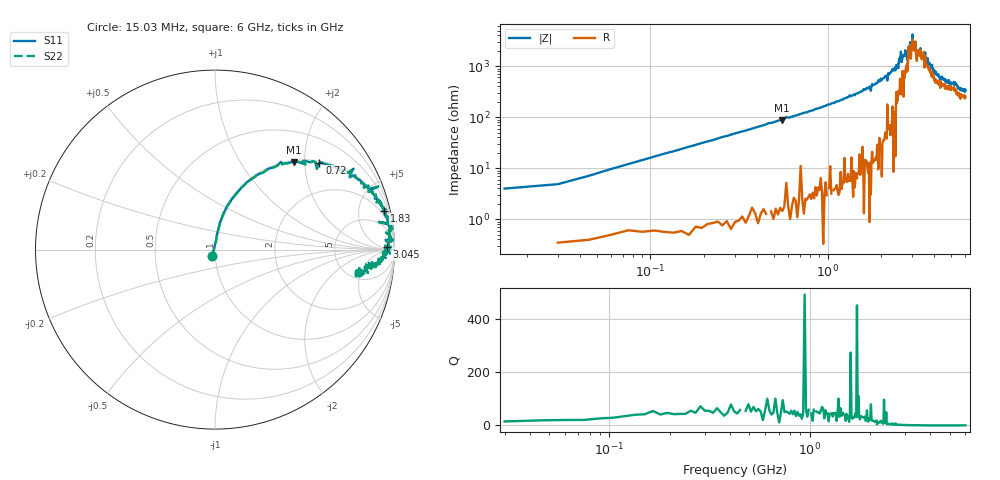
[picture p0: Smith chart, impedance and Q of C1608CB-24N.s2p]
!	Network	Analyzer	HP8753E.07.74:	Oct	30	2002	Serial	No.	JP38451487
!	Hewlett-Packard
!	28	Aug	2009	16:01:57
!	Frequency	S11	S21	S12	S22
#	HZ	S	RI	R	50
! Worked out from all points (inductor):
!   400 points, 15.03 MHz to 6 GHz, reference 50 ohm
!   read as one part in series: L = 25.5 nH near 45.03 MHz
!   highest Q = 56 at 555 MHz (marker M1), where L = 25.3 nH
!   self-resonance near 3.06 GHz
!   S11 on the Smith chart (normalised r, x): 15.03 MHz: 0.97, -0.07; 720 MHz: 1.05, +2.37; 1.83 GHz: 1.28, +8.66; 3.045 GHz: 42, +14; 6 GHz: 6.02, -4.38
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1.502992e7  -0.0163 -0.0363  1.02 0.0363  1.02 0.0363  -0.0163 -0.0363
9.002955e7  0.0255 0.14  0.974 -0.14  0.974 -0.14  0.0255 0.14
1.95029e8  0.0937 0.281  0.906 -0.281  0.906 -0.281  0.0937 0.281
5.550272e8  0.438 0.488  0.562 -0.488  0.562 -0.488  0.438 0.488
7.200264e8  0.582 0.483  0.418 -0.483  0.418 -0.483  0.582 0.483
1.020025e9  0.753 0.42  0.247 -0.42  0.247 -0.42  0.753 0.42
1.830021e9  0.943 0.216  0.0568 -0.216  0.0568 -0.216  0.943 0.216
2.01002e9  0.957 0.18  0.0427 -0.18  0.0427 -0.18  0.957 0.18
2.505017e9  0.953 0.0942  0.047 -0.0942  0.047 -0.0942  0.953 0.0942
2.595017e9  0.99 0.0501  0.00995 -0.0501  0.00995 -0.0501  0.99 0.0501
2.625017e9  0.971 0.075  0.0293 -0.075  0.0293 -0.075  0.971 0.075
2.835016e9  0.95 0.0545  0.0504 -0.0545  0.0504 -0.0545  0.95 0.0545
2.865016e9  0.962 0.0115  0.0382 -0.0115  0.0382 -0.0115  0.962 0.0115
3.000015e9  0.964 0.017  0.0364 -0.017  0.0364 -0.017  0.964 0.017
3.015015e9  0.981 0.014  0.0188 -0.014  0.0188 -0.014  0.981 0.014
3.045015e9  0.958 0.0139  0.042 -0.0139  0.042 -0.0139  0.958 0.0139
3.135014e9  0.969 0.00607  0.0312 -0.00607  0.0312 -0.00607  0.969 0.00607
3.195014e9  0.936 -0.0248  0.0636 0.0248  0.0636 0.0248  0.936 -0.0248
3.345013e9  0.96 -0.0145  0.0399 0.0145  0.0399 0.0145  0.96 -0.0145
4.00501e9  0.919 -0.0803  0.0813 0.0803  0.0813 0.0803  0.919 -0.0803
5.010005e9  0.843 -0.0908  0.157 0.0908  0.157 0.0908  0.843 -0.0908
6e9  0.795 -0.128  0.205 0.128  0.205 0.128  0.795 -0.128
